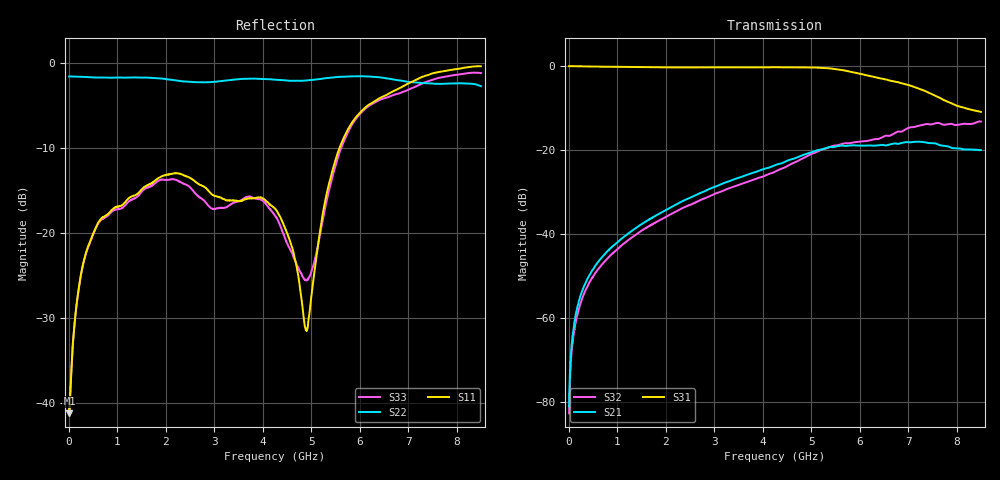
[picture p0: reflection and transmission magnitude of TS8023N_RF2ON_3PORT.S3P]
!Agilent Technologies,E5071C,MY46522130,B.12.04
!Date: Thu Jul 17 20:35:55 2025
!Data & Calibration Information:
!Freq	S11:SOLT3(ON)	S13:SOLT3(ON)	S14:SOLT3(ON)
!	S31:SOLT3(ON)	S33:SOLT3(ON)	S34:SOLT3(ON)
!	S41:SOLT3(ON)	S43:SOLT3(ON)	S44:SOLT3(ON)
!PortZ  Port1:50+j0  Port3:50+j0  Port4:50+j0
!Above PortZ is port z conversion or system Z0 setting when saving the data.
!When reading, reference impedance value at option line is always used.
# Hz S dB R 50
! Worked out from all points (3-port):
!   1601 points, 10 MHz to 8.5 GHz, reference 50 ohm
!   strongest paths, dB at 10 MHz, 2.132 GHz, 4.255 GHz, 6.378 GHz, 8.5 GHz:
!     S31: -0.1, -0.4, -0.4, -2.9, -11.0
!     S21: -81.0, -33.5, -23.6, -18.9, -20.1
!     S32: -82.6, -35.1, -25.2, -17.4, -13.3
!   lowest |S11| = -41.2 dB at 15.31 MHz (marker M1), VSWR 1.02, Z = 50.8 - j0.29 ohm
!   |S11| at or under -10 dB: start of sweep to 5.583 GHz
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1e7  -40.75 -10.2  -80.64 57.4  -0.12 -0.2
     -80.96 60.3  -1.59 179.8  -80.84 45.7
     -0.12 -0.2  -82.62 46.8  -40.53 -9.3
1.530625e7  -41.16 -19.0  -77.99 67.5  -0.12 -0.3
            -78.05 67.5  -1.58 179.7  -78.43 52.9
            -0.12 -0.3  -78.65 66.9  -40.82 -18.5
2.2225e8  -25.95 -87.5  -55.55 89.1  -0.15 -4.7
          -55.64 88.1  -1.61 177.7  -57.40 88.7
          -0.15 -4.7  -57.39 88.6  -26.02 -86.6
7.847125e8  -17.84 -101.6  -44.24 92.4  -0.25 -16.2
            -44.27 92.7  -1.71 169.0  -46.02 91.5
            -0.25 -16.2  -46.03 91.4  -18.02 -104.4
4.255e9  -17.11 -121.7  -23.79 61.4  -0.39 -89.7
         -23.64 61.6  -1.96 101.4  -25.07 63.9
         -0.37 -89.8  -25.20 63.6  -17.92 127.2
4.902362e9  -31.37 -174.3  -20.97 47.3  -0.40 -107.5
            -20.99 47.1  -2.05 87.5  -21.62 52.7
            -0.40 -107.6  -21.60 52.6  -25.47 114.5
5.321556e9  -15.30 115.5  -19.61 32.2  -0.57 -121.4
            -19.51 33.3  -1.77 78.3  -19.52 39.8
            -0.58 -121.4  -19.63 39.0  -16.16 151.8
5.846875e9  -6.96 104.3  -19.12 13.5  -1.51 -139.9
            -18.93 14.1  -1.57 76.1  -18.10 21.7
            -1.53 -140.1  -18.30 21.6  -7.20 147.5
7.417525e9  -1.40 53.5  -18.14 -26.2  -6.44 176.0
            -18.37 -26.2  -2.39 67.4  -14.09 -20.8
            -6.38 176.3  -13.90 -21.9  -2.12 110.3
8.5e9  -0.38 57.1  -19.98 -38.6  -10.94 171.8
       -20.06 -37.0  -2.72 61.0  -13.20 -38.7
       -10.98 171.9  -13.28 -39.8  -1.17 95.5
